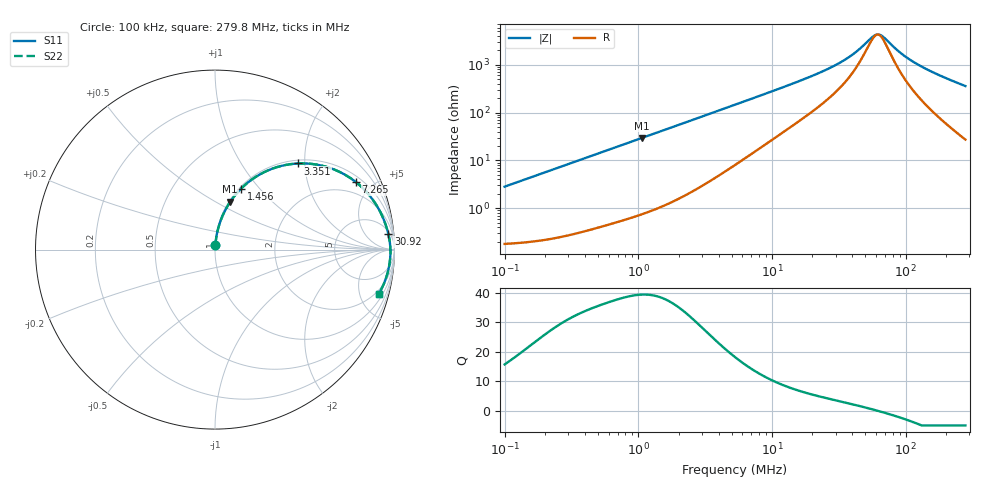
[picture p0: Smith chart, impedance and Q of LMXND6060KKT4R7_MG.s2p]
! LMXND6060KKT4R7_MG  S-PARAMETER MODEL  ( General Type )
! Model Generated by TAIYO YUDEN Corporation (http://www.ty-top.com)
! Version 1.0
! TAIYO YUDEN Control No. 191023NI43SB-FBB
! Copyright(c) 2019 TAIYO YUDEN CO.,LTD. All Rights Reserved.
! Product Description (link to TY-COMPAS)
! https://ds.yuden.co.jp/TYCOMPAS/or/detail?pn=LMXND6060KKT4R7MMG&u=M
! Products Name : Inductors
! Characteristics :
!  Inductance : 4.7 uH , SRF(min) : 36 MHz , DC Resistance(max) : 0.198 Ohm
!  Rated Current : Saturation :1300 mA , Temp Rise : 1400 mA
!  Case Size : 6.0 x 6.0 / 0.236 x 0.236 [mm/inch] , Thickness : 1 / 0.039 [mm/inch]
!  (Conditions: Temperature = 25 degC , DC Bias Current/Voltage = 0A / 0V)
! External Node Assignments :
!  1  o---GGG---o  2
! GND o---------o GND
! Frequency Range : 0.1MHz  -  279.750408MHz  [ 402 STEP ]
# MHz S RI R 50
! Freq[MHz].  S11 Real  S11 Imag  S21 Real  S21 Imag  S12 Real  S12 Imag  S22 Real  S22 Imag
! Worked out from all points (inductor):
!   401 points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, 100 kHz to 279.8 MHz, reference 50 ohm
!   read as one part in series: L = 4.48 uH near 104 kHz
!   highest Q = 39.5 at 1.06 MHz (marker M1), where L = 4.41 uH
!   self-resonance near 61.61 MHz
!   S11 on the Smith chart (normalised r, x): 100 kHz: 1.00, +0.06; 1.456 MHz: 1.02, +0.81; 3.351 MHz: 1.07, +1.85; 7.265 MHz: 1.29, +4.02; 30.92 MHz: 7, +20; 279.8 MHz: 1.55, -7.17
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0.1  0.00258 0.0281  0.9974 -0.0281  0.9974 -0.0281  0.00258 0.0281
0.377863  0.0141 0.104  0.9859 -0.104  0.9859 -0.104  0.0141 0.104
0.645641  0.0356 0.1725  0.9644 -0.1725  0.9644 -0.1725  0.0356 0.1725
1.060265  0.0852 0.2668  0.9148 -0.2668  0.9148 -0.2668  0.0852 0.2668
1.427803  0.1413 0.3357  0.8587 -0.3357  0.8587 -0.3357  0.1413 0.3357
1.456415  0.146 0.3404  0.854 -0.3404  0.854 -0.3404  0.146 0.3404
2.165826  0.2696 0.4293  0.7304 -0.4293  0.7304 -0.4293  0.2696 0.4293
3.351167  0.4629 0.4799  0.5371 -0.4799  0.5371 -0.4799  0.4629 0.4799
5.289144  0.6727 0.4426  0.3273 -0.4426  0.3273 -0.4426  0.6727 0.4426
7.265344  0.7858 0.3756  0.2142 -0.3756  0.2142 -0.3756  0.7858 0.3756
11.46689  0.8877 0.2658  0.1123 -0.2658  0.1123 -0.2658  0.8877 0.2658
19.9857  0.9454 0.1538  0.0546 -0.1538  0.0546 -0.1538  0.9454 0.1538
30.92373  0.9657 0.0868  0.0343 -0.0868  0.0343 -0.0868  0.9657 0.0868
40.82525  0.9727 0.0503  0.0273 -0.0503  0.0273 -0.0503  0.9727 0.0503
54.97721  0.9767 0.0138  0.0233 -0.0138  0.0233 -0.0138  0.9767 0.0138
59.51829  0.9772 0.00418  0.0228 -0.00418  0.0228 -0.00418  0.9772 0.00418
65.72568  0.9775 -0.00785  0.0225 0.00785  0.0225 0.00785  0.9775 -0.00785
75.51853  0.9774 -0.0249  0.0226 0.0249  0.0226 0.0249  0.9774 -0.0249
95.82011  0.9754 -0.0556  0.0246 0.0556  0.0246 0.0556  0.9754 -0.0556
124.0157  0.9702 -0.0922  0.0298 0.0922  0.0298 0.0922  0.9702 -0.0922
180.8  0.9539 -0.1554  0.0461 0.1554  0.0461 0.1554  0.9539 -0.1554
279.7504  0.912 -0.2478  0.088 0.2478  0.088 0.2478  0.912 -0.2478
